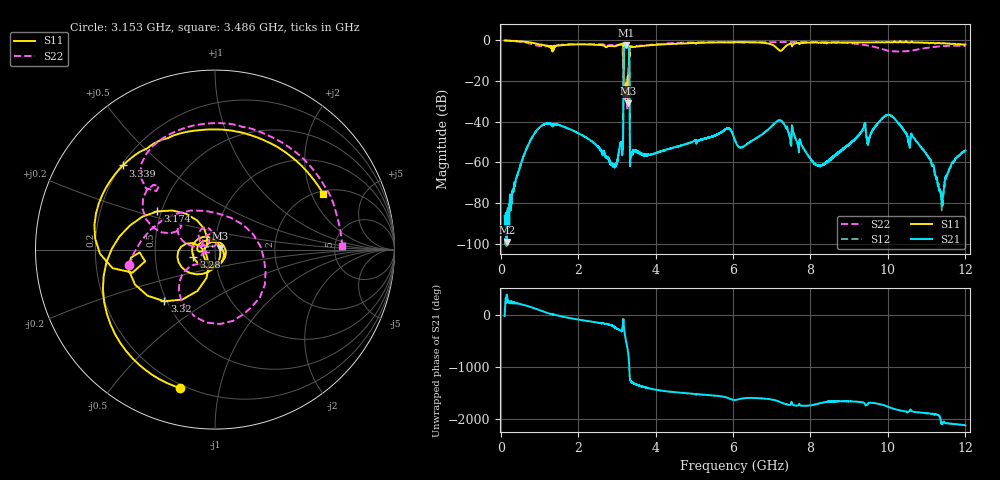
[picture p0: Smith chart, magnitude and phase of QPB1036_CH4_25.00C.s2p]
! TDS: K:\Engsetup\Winsaw\QPB1036_ALL
! Channel 1
! Ports=1 2
! seg 1=100.000000 1100.000000 101
! seg 2=1101.000000 1501.000000 401
! seg 3=1502.000000 2502.000000 101
! seg 4=2503.000000 3803.000000 1301
! seg 5=3804.000000 5004.000000 121
! seg 6=5005.000000 6005.000000 1001
! seg 7=6006.000000 8406.000000 241
! seg 8=8407.000000 10607.000000 2201
! seg 9=10608.000000 12008.000000 141
! Points=5609
! FailCode=0
! Topology=ALL_SE(12)
!VNA Cal loaded =QPB1036_ALL_25C
!PS1(V)= 5.000
!PS(mA)= 0.500
!PS2(V)= 1.170
!PS(mA)= -0.100
!PS3(V)= 0.630
!PS(mA)= 0.100
!PS4(V)= 0.630
!PS(mA)= -0.100
!Temp (C)= 25.00
# MHz S DB R 50
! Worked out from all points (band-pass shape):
!   5609 points, 100 MHz to 12.01 GHz, reference 50 ohm
!   highest |S21| = -2.71 dB at 3.239 GHz (marker M1); lowest = -98.9 dB at 160 MHz (marker M2)
!   |S21| within 3 dB of the highest: 3.184 GHz to 3.317 GHz (133.1 MHz wide, 4.09 % of centre)
!   lowest |S11| = -31.1 dB at 3.296 GHz (marker M3), VSWR 1.06, Z = 52.7 + j1.03 ohm
!   |S11| at or under -10 dB: 3.175 GHz to 3.319 GHz (143.8 MHz wide, 4.43 % of centre)
!   |S22| runs from -34.1 to -0.3 dB; largest |S21 - S12| = 0.007
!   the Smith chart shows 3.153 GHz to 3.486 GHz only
!   S11 on the Smith chart (normalised r, x): 3.153 GHz: 0.18, -0.76; 3.174 GHz: 0.48, +0.24; 3.28 GHz: 0.78, -0.06; 3.32 GHz: 0.48, -0.33; 3.339 GHz: 0.21, +0.37; 3.486 GHz: 2.13, +2.45
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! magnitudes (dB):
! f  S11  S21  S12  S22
! 100 MHz  -0.3  -86.3  -100.5  -0.3
! 160 MHz  -0.4  -98.9  -85.5  -0.4
! 1.124 GHz  -2.8  -41.4  -41.4  -3.2
! 2.092 GHz  -2.2  -46.6  -46.6  -2.0
! 2.942 GHz  -3.2  -61.4  -61.6  -3.0
! 3.153 GHz  -2.0  -52.7  -52.7  -6.3
! 3.174 GHz  -8.3  -15.8  -15.8  -7.8
! 3.2 GHz  -25.2  -3.5  -3.5  -20.0
! 3.239 GHz  -24.3  -2.7  -2.7  -22.2
! 3.28 GHz  -18.0  -3.1  -3.0  -19.3
! 3.296 GHz  -31.1  -3.5  -3.4  -22.1
! 3.32 GHz  -7.9  -7.5  -7.5  -7.6
! 3.339 GHz  -3.2  -59.5  -59.2  -3.1
! 3.364 GHz  -3.5  -56.8  -56.7  -3.1
! 3.486 GHz  -3.4  -54.6  -54.6  -3.0
! 4.074 GHz  -2.3  -54.9  -54.9  -2.1
! 6.056 GHz  -1.1  -49.3  -49.2  -1.2
! 7.176 GHz  -4.8  -39.4  -39.5  -1.1
! 8.046 GHz  -1.3  -59.5  -59.0  -1.0
! 10.02 GHz  -1.0  -36.6  -36.7  -5.3
! 11.33 GHz  -1.5  -73.8  -72.6  -3.2
! 12.01 GHz  -2.3  -54.2  -54.2  -3.0
